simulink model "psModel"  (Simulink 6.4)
settings: Solver=ode113  StartTime=psSimStruct.psSimPar.tStart  StopTime=psSimStruct.psSimPar.tStop  MaxStep=psSimStruct.psSimPar.maxStep  RelTol=psSimStruct.psSimPar.relTol
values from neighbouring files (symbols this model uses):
  psSimStruct = []    [psStartUp.m]
undefined symbols (not defined in the file or in its folder): psDVolume, psVolume

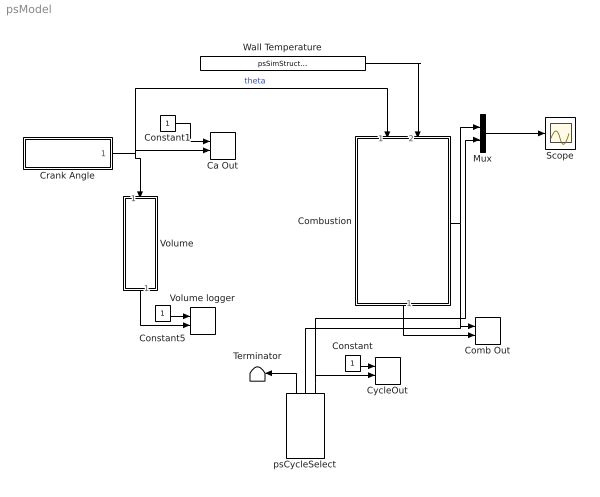
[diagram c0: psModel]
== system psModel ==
  Ca Out : M-S-Function  FunctionName=psToWorkspace  Parameters=1,int16('theta'),1
  Comb Out : M-S-Function  FunctionName=psToWorkspace  Parameters=9+2*psSimStruct.psThermProp.K,int16('pcb Vb Tb Vu Tu'),1
  Combustion : Subsystem  Orientation=down  TreatAsAtomicUnit=on
  Constant : Constant
  Constant1 : Constant
  Constant5 : Constant
  Crank Angle : Subsystem
  CycleOut : M-S-Function  FunctionName=psToWorkspace  Parameters=1,int16('phase'),1
  Mux : Mux  Inputs=2
  Scope : Scope
  Terminator : Terminator
  Volume : Subsystem  Orientation=down
  Volume logger : M-S-Function  FunctionName=psToWorkspace  Parameters=1,int16('V'),1
  Wall Temperature : Constant  Value=psSimStruct.psModel.T_Wall
  psCycleSelect : M-S-Function  Orientation=up  FunctionName=psCycleSelect  Parameters=caOffset  mask{caOffset=0}
      mask prompts: caOffset "caOffset [rad]"
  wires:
  Volume/1(V) -> Volume logger/2
  Constant5/1 -> Volume logger/1
  Crank Angle/1(theta [rad]) -> Ca Out/2, Volume/1(theta in), Combustion/1(theta)  "theta"
  Wall Temperature/1 -> Combustion/2(Wall Temperature)
  Combustion/1(IntOut) -> Comb Out/2
  Constant1/1 -> Ca Out/1
  Constant/1 -> CycleOut/1
  psCycleSelect/1 -> Terminator/1
  psCycleSelect/2 -> Comb Out/1, Combustion/Enable, Mux/1
  Mux/1 -> Scope/1
  psCycleSelect/3 -> CycleOut/2, Mux/2

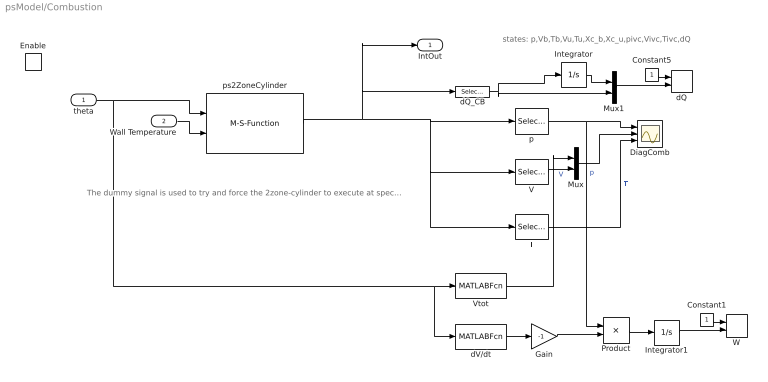
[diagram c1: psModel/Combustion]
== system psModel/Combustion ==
  note: states: p,Vb,Tb,Vu,Tu,Xc_b,Xc_u,pivc,Vivc,Tivc,dQ
  note: The dummy signal is used to try and force the 2zone-cylinder to execute at specific events
  theta : Inport
  Wall Temperature : Inport  Port=2
  Enable : EnablePort  Orientation=left  StatesWhenEnabling=reset
  Constant1 : Constant
  Constant5 : Constant
  DiagComb : Scope  NumInputPorts=3
  Gain : Gain  Gain=-1
  Integrator : Integrator
  Integrator1 : Integrator
  Mux : Mux  Inputs=2
  Mux1 : Mux  Inputs=2
  Product : Product
  T : Selector  Elements=[3 5]  Rows=[3 5]  OutputPortSize=[(-2)]
  V : Selector  Elements=[2 4]  Rows=[2 4]  OutputPortSize=[(-2)]
  Vtot : MATLABFcn  MATLABFcn=psVolume(u(1))  OutputDimensions=1
  W : M-S-Function  FunctionName=psToWorkspace  Parameters=1,int16('W'),1
  dQ : M-S-Function  FunctionName=psToWorkspace  Parameters=2,int16('Q dQ'),1
  dQ_CB : Selector  Elements=[psSimStruct.psThermProp.K*2+9]  Rows=[psSimStruct.psThermProp.K*2+9]  OutputPortSize=[(-2)]
  dV/dt : MATLABFcn  MATLABFcn=psDVolume(u(1))*psSimStruct.psSimPar.w  OutputDimensions=1
  p : Selector  Elements=[1]  Rows=[1]  OutputPortSize=[(-2)]
  ps2ZoneCylinder : M-S-Function  FunctionName=ps2ZoneCylinder  Parameters=0,1
  IntOut : Outport
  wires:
  dQ_CB/1 -> Integrator/1, Mux1/2
  Constant5/1 -> dQ/1
  ps2ZoneCylinder/1 -> dQ_CB/1, IntOut/1, p/1, V/1, T/1
  p/1 -> DiagComb/1, Product/1  "p"
  T/1 -> DiagComb/3  "T"
  V/1 -> Mux/2  "V"
  Mux/1 -> DiagComb/2
  Vtot/1 -> Mux/1
  theta/1 -> ps2ZoneCylinder/1, Vtot/1, dV/dt/1
  Wall Temperature/1 -> ps2ZoneCylinder/2
  Integrator/1 -> Mux1/1
  Mux1/1 -> dQ/2
  dV/dt/1 -> Gain/1
  Product/1 -> Integrator1/1
  Constant1/1 -> W/1
  Integrator1/1 -> W/2
  Gain/1 -> Product/2

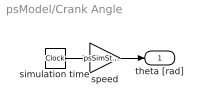
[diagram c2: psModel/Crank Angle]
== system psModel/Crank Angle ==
  simulation time : Clock
  speed : Gain  Gain=psSimStruct.psSimPar.w
  theta [rad] : Outport
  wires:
  speed/1 -> theta [rad]/1
  simulation time/1 -> speed/1

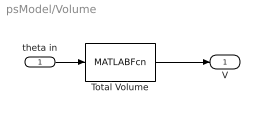
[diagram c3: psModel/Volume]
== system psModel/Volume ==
  theta in : Inport
  Total Volume : MATLABFcn  Description=|  MATLABFcn=psVolume(u(1))  OutputDimensions=1
      | [u] = psValve(CA)                                   
      | Calculates the valve states. u = [u1 u2]', where u1  
      | is the intake valve and u2 the outlet valve.         
      | u1, u2 = 1 means fully open, u1, u2 = 0 means closed.
  V : Outport
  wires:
  Total Volume/1 -> V/1
  theta in/1 -> Total Volume/1
